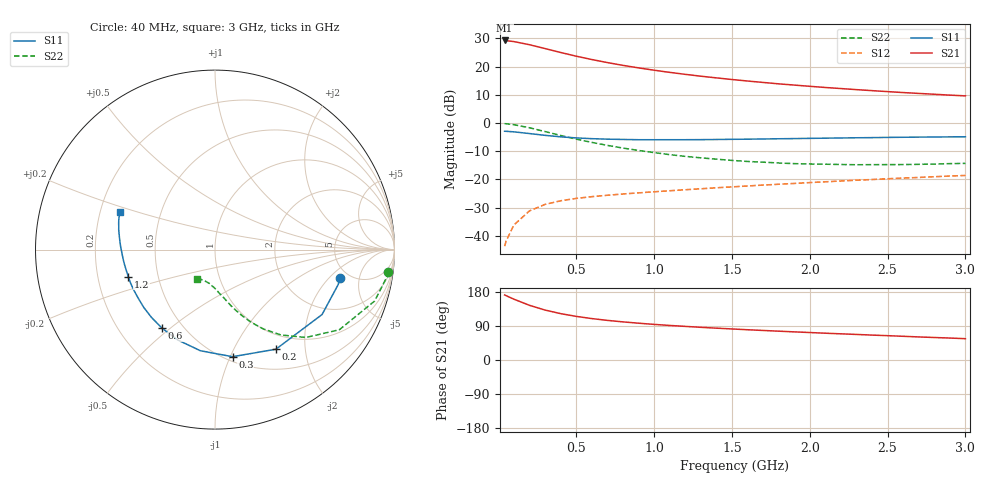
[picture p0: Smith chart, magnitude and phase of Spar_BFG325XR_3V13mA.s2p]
! Filename: 313BFG325XR.s2p
! Title: BFG325XR,RN20042071,Lot:TT3899C,B:Y13641,Sl.:1
! Bias: VCE=2.999V; IC=12.89mA;
! Company: NXP Semiconductors NL
! User: Q&R DSC-N
! Measure time: 29 Mar 2004 / 13:40:20
#  MHz  S  MA  R 50
! Freq  S11  S21  S12  S22  :
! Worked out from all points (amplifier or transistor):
!   32 points, 40 MHz to 3 GHz, reference 50 ohm
!   highest |S21| = 29.3 dB at 40 MHz (marker M1)
!   |S21| within 3 dB of that: start of sweep to 309 MHz
!   unconditionally stable (mu >= 1): 1.919 GHz to end of sweep
!   at 400 MHz: K = 0.38, MSG = 26.3 dB, |S12| = -27.6 dB
!   at 1.5 GHz: K = 0.93, MSG = 19.0 dB, |S12| = -22.6 dB
!   at 3 GHz: K = 1.05, MAG = 12.7 dB, |S12| = -18.6 dB
!   S11 on the Smith chart (normalised r, x): 40 MHz: 4.20, -2.72; 200 MHz: 0.78, -1.49; 300 MHz: 0.54, -1.02; 600 MHz: 0.39, -0.47; 1.2 GHz: 0.33, -0.14; 3 GHz: 0.28, +0.18
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40  0.7156 -12.8  29.06 171.7  0.006567 83.8  0.974 -7.2
50  0.7133 -15.9  28.87 169.7  0.008151 82.4  0.9698 -9.1
100  0.6977 -31.2  27.76 160.4  0.01563 75.3  0.9343 -17.9
200  0.6504 -58.5  24.42 144.2  0.02775 64.0  0.8242 -32.8
300  0.6047 -80.7  20.87 131.8  0.03612 56.2  0.7047 -44.0
400  0.5692 -98.2  17.78 122.4  0.04188 51.2  0.6011 -52.3
500  0.5446 -112.4  15.3 115.1  0.04614 48.4  0.5185 -58.5
600  0.5281 -123.8  13.35 109.3  0.04952 46.7  0.4537 -63.5
700  0.5178 -133.1  11.79 104.5  0.05245 45.9  0.4017 -67.5
800  0.5112 -140.9  10.52 100.6  0.05525 45.6  0.3599 -70.9
900  0.5063 -147.5  9.493 97.1  0.05781 45.7  0.3266 -74.0
1000  0.5055 -153.3  8.631 94.0  0.0604 45.9  0.2991 -76.7
1100  0.5061 -158.3  7.907 91.2  0.06306 46.2  0.2753 -79.3
1200  0.5063 -162.7  7.291 88.7  0.06569 46.6  0.2564 -82.2
1300  0.5076 -166.8  6.762 86.2  0.06835 47.0  0.2416 -84.8
1400  0.5107 -170.3  6.314 84.0  0.07119 47.4  0.2288 -87.1
1600  0.5171 -176.5  5.553 79.8  0.07651 48.2  0.2084 -92.4
1800  0.5259 178.2  4.949 76.1  0.08217 48.9  0.1958 -97.2
2100  0.5389 171.8  4.263 70.7  0.09084 49.4  0.1861 -104.6
2400  0.5512 166.6  3.75 65.7  0.09962 49.7  0.1828 -111.3
2600  0.5593 163.6  3.467 62.6  0.1058 49.8  0.1836 -115.1
3000  0.57 158.2  3.025 56.3  0.1177 49.0  0.1925 -122.2
